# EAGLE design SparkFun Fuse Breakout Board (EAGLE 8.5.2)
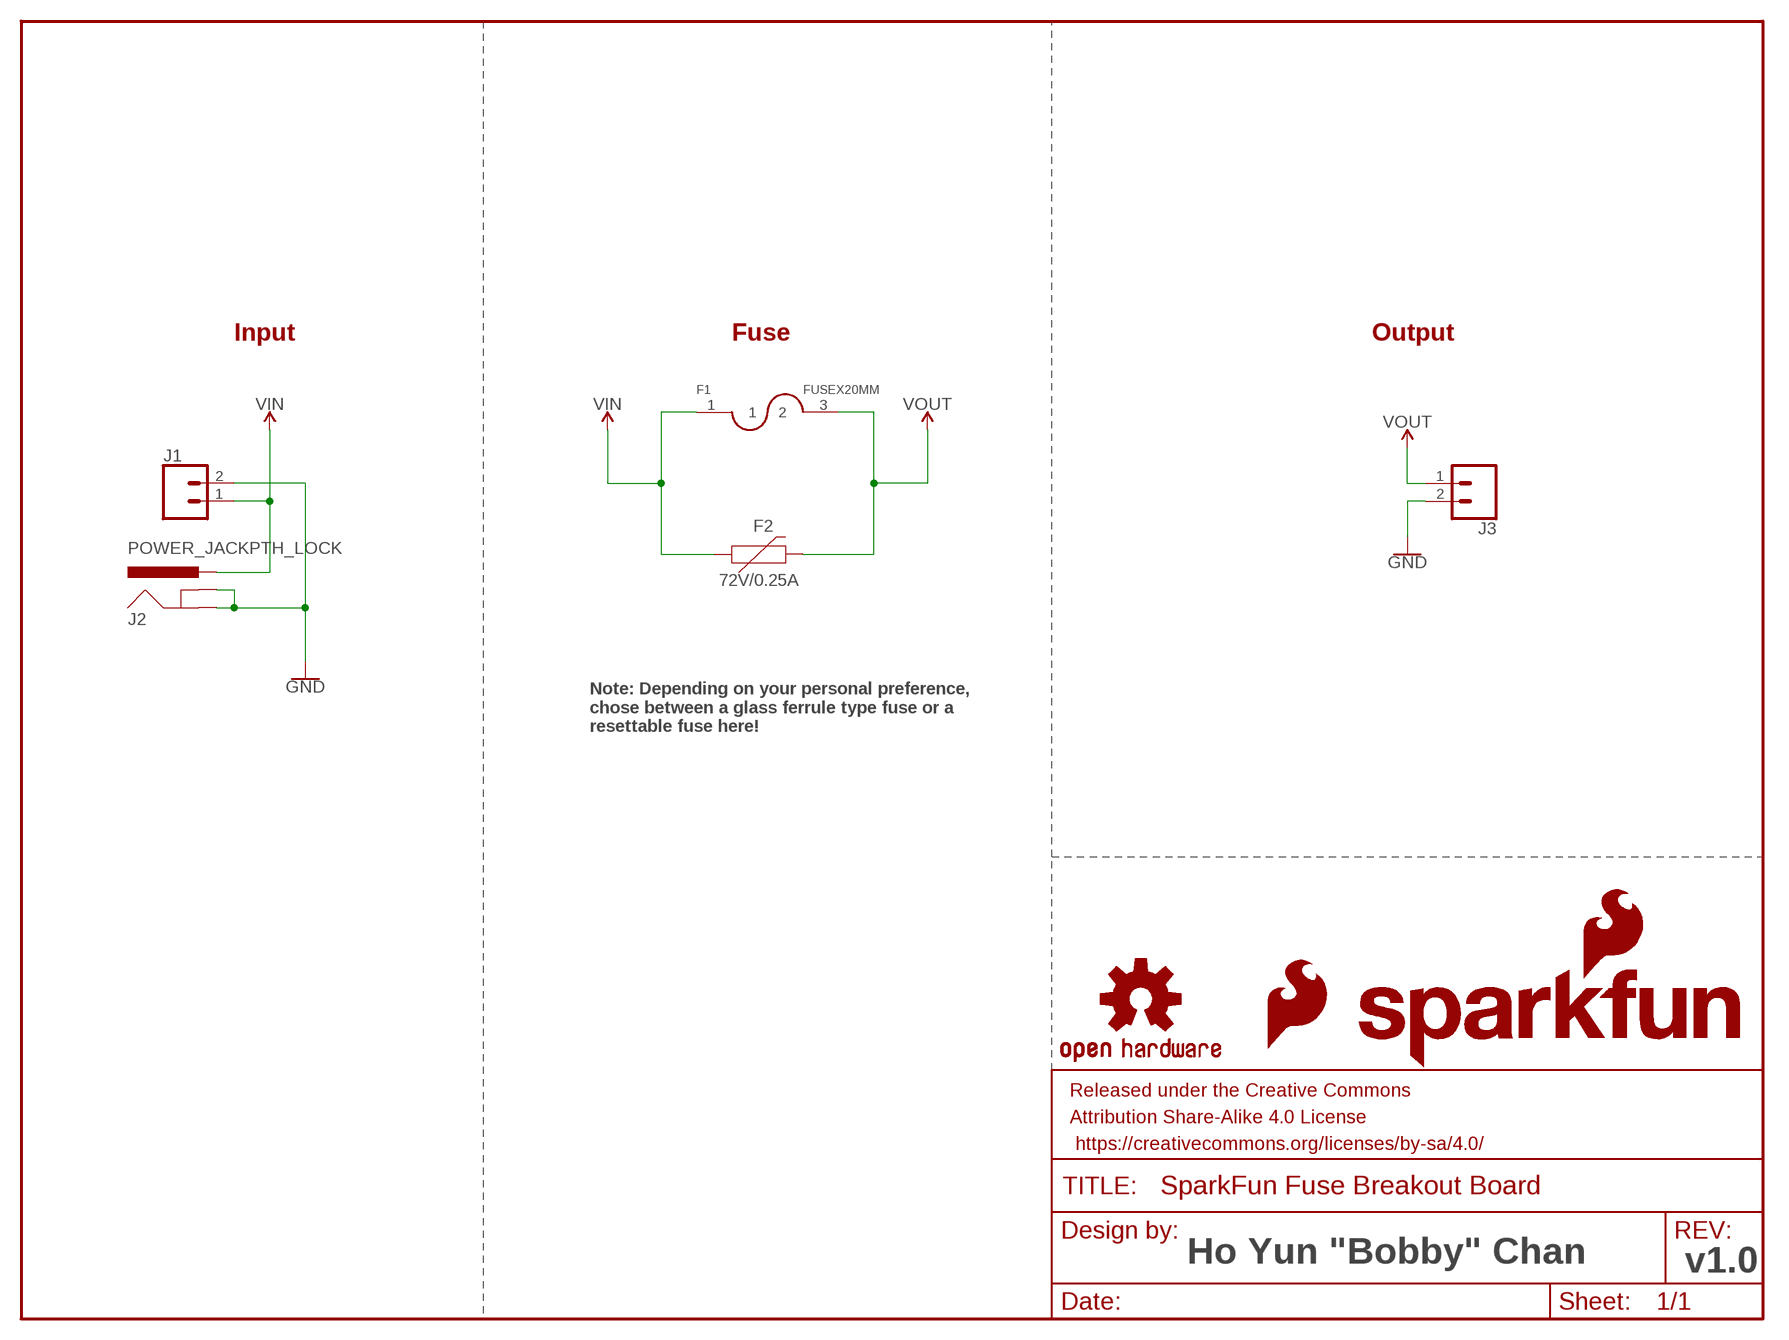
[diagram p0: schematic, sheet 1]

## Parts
F1  FUSEX20MM  [FUSE_5MM]
F2  72V/0.25A  PPTC_PTH  [PTH]
FRAME1  FRAME-LETTER  [CREATIVE_COMMONS]
J1  CONN_025MM  [SCREWTERMINAL-5MM-2]
J2  POWER_JACKPTH_LOCK  [POWER_JACK_PTH_LOCK]
J3  CONN_025MM  [SCREWTERMINAL-5MM-2]
LOGO1  SFE_LOGO_NAME_FLAME.1_INCH  [SFE_LOGO_NAME_FLAME_.1]
LOGO2  SFE_LOGO_FLAME.1_INCH  [SFE_LOGO_FLAME_.1]
LOGO3  OSHW-LOGOMINI  [OSHW-LOGO-MINI]

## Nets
GND: J1.2 J2.GND J2.GNDBREAK J3.2
VIN: F1.1 F2.P$1 J1.1 J2.PWR
VOUT: F1.3 F2.P$2 J3.1

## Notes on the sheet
- Input | Fuse | Output
- Note: Depending on your personal preference,
  chose between a glass ferrule type fuse or a
  resettable fuse here!
- Ho Yun "Bobby" Chan | v1.0

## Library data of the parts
F1 = SparkFun:FUSE
F2 = SparkFun-Fuses:PPTC: Resettable Fuse PPTC; PROD_ID: RES-08490
FRAME1 = SparkFun-Aesthetics:FRAME-LETTER: Schematic Frame - Letter
J1 J3 = SparkFun-Connectors:CONN_02: Multi connection point. Often used as Generic Header-pin footprint for 0.1 inch spaced/style header connections; SF_SKU: PRT-08432
J2 = SparkFun-Connectors:POWER_JACK: Power Jack Connector This is the standard 5.5mm barrel jack for power. The PTH is the most common, proven, reliable, footprint. The Slot footprint only works if the mill layer is transmitted to the PCB fab house so be warned. Here are the connectors we sell at SparkFun: DC Barrel Power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; PROD_ID: CONN-08197; SF_ID: PRT-00119
LOGO1 = SparkFun-Aesthetics:SFE_LOGO_NAME_FLAME: SparkFun Font Logo w/ Flame
LOGO2 = SparkFun-Aesthetics:SFE_LOGO_FLAME: SparkFun Flame Logo
LOGO3 = SparkFun-Aesthetics:OSHW-LOGO: Open-Source Hardware (OSHW) Logo

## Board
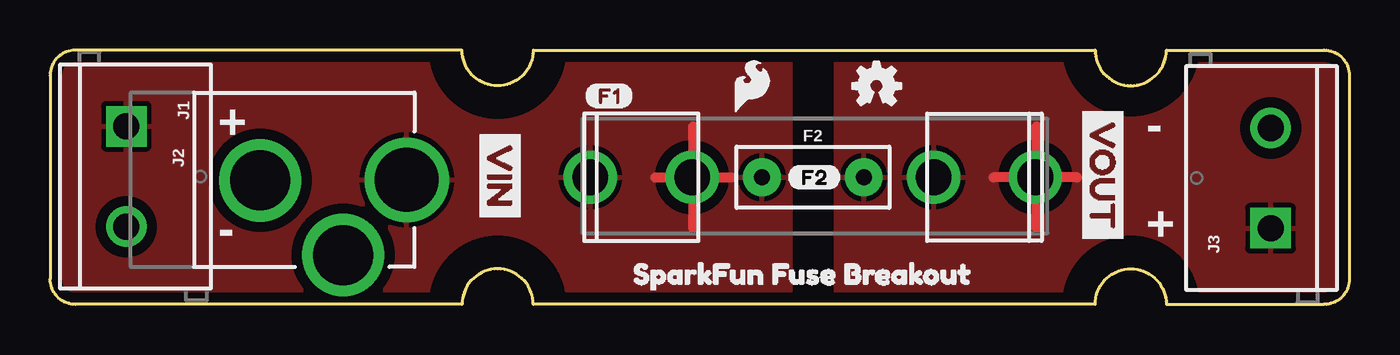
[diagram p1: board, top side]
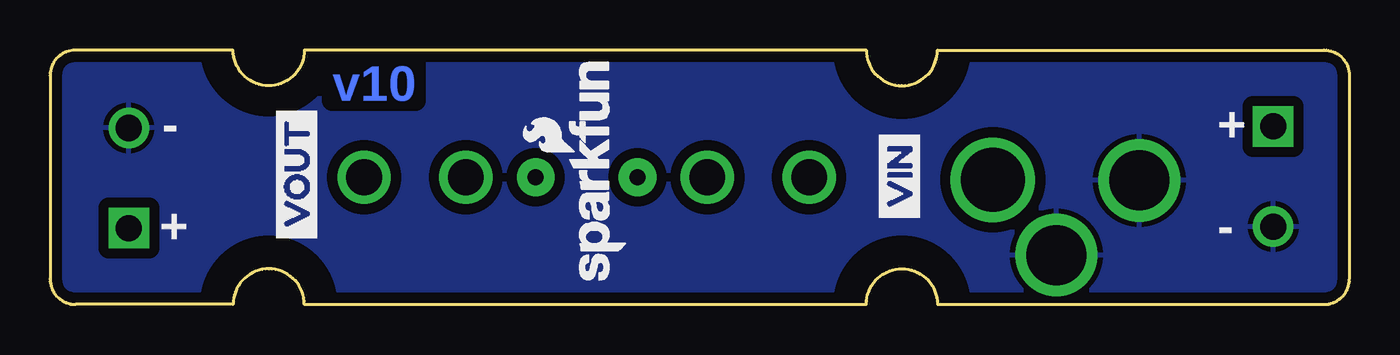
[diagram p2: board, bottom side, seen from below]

Size 64.9 x 12.7 mm. Coordinates in mm from the lower left corner, seen from the top.
Outline: 24.13,12.7 52.2,12.7 arc90 53.98,10.92 arc90 55.75,12.7 63.63,12.7 arc-90 64.9,11.43 64.9,1.27 arc-90 63.63,0 55.75,0 arc90 53.98,1.78 arc90 52.2,0 24.13,0 arc90 22.35,1.78 arc90 20.57,0 1.27,0 arc-90 0,1.27 0,11.43 arc-90 1.27,12.7 20.57,12.7 arc90 22.35,10.92 arc90 24.13,12.7
Copper layers (1*16): Top 0.035mm / dielectric 1.5mm / Bottom 0.035mm
Design rules "SparkFun-2-layer-STANDARD": minimum track width 10mil, minimum drill 20mil, track to track 10mil, track to pad 8mil, pad to pad 8mil, via to via 10mil, smd to smd 8mil, copper to edge 8mil, drill to drill 8mil, minimum pad ring 10mil, minimum via ring 10mil, stop-mask expansion 4mil, vias tented up to drill 25mil, thermal gap 10mil
tRestrict: area 19.5,-2.8 to 25.2,2.8; area 19.5,9.9 to 25.2,15.5; area 51.1,10 to 56.8,15.7; area 51.1,-2.8 to 56.8,2.8
bRestrict: area 19.5,9.9 to 25.2,15.5; area 19.5,-2.8 to 25.2,2.8; area 51.1,10 to 56.8,15.7; area 51.1,-2.8 to 56.8,2.8

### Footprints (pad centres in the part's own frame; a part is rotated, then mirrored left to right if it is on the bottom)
FUSE_5MM = drill 1.778: 1 0,-11.113; 2 0,-6.032; 3 0,6.032; 4 0,11.113
PTH = drill 0.8 pad 1.88: P$1 -2.54,0; P$2 2.54,0
SCREWTERMINAL-5MM-2 = drill 1.3 pad 2.032 square: 1 0,0 | drill 1.3 pad 2.032: 2 5,0
POWER_JACK_PTH_LOCK = drill 2.997 pad 4.115: GND 0.025,6.557; GNDBREAK 3.762,10.7 | drill 3.2 pad 4.115: PWR 0,13.878

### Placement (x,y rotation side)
F1  38.1,6.35 270 top
F2  38.1,6.35 0 top
FRAME1  not placed on the board
J1  3.81,8.89 270 top
J2  3.94,6.22 270 top
J3  60.96,3.81 90 top
LOGO1  36.07,0.76 90 bottom
LOGO2  33.91,9.27 0 top
LOGO3  41.27,10.92 0 top
U$1  [VIN0]  22.48,9.14 270 top
U$2  [VOUT0]  52.58,10.29 270 top
U$3  [VOUT0]  52.58,2.67 90 bottom
U$4  [VIN0]  22.48,3.68 90 bottom
U$11  [SPARKFUN_FUSE_BREAKOUT0]  28.19,1.52 0 top
U$28  [F10]  26.67,10.41 0 top
U$29  [F20]  36.83,6.35 0 top

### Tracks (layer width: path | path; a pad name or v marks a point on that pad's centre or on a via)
GND
  pour Bottom (isolate 0.508): 52.2,12.7 24.13,12.7 arc-90 22.35,10.92 arc-90 20.57,12.7 1.27,12.7 arc90 0,11.43 0,1.27 arc90 1.27,0 20.57,0 arc-90 22.35,1.78 arc-90 24.13,0 52.2,0 arc-90 53.98,1.78 arc-90 55.75,0 63.63,0 arc90 64.9,1.27 64.9,11.43 arc90 63.63,12.7 55.75,12.7 arc-90 53.98,10.92 arc-90
VIN
  Top 0.508: 32.13,3.81 32.13,8.89 | 30.23,6.35 34.04,6.35
  pour Top (isolate 0.508): 36.96,0 1.27,0 arc-90 0,1.27 0,11.43 arc-90 1.27,12.7 36.96,12.7
VOUT
  Top 0.508: 51.31,6.35 47.12,6.35 | 49.28,3.81 49.28,8.89
  pour Top (isolate 0.508): 39.24,0 63.5,0 arc90 64.77,1.27 64.77,11.43 arc90 63.5,12.7 39.24,12.7

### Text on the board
Bottom: v10
tPlace: + | - | - | +
bPlace: + | - | - | +
Measures: Dimensions are given in inches.
tDocu: Ho Yun "Bobby" Chan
